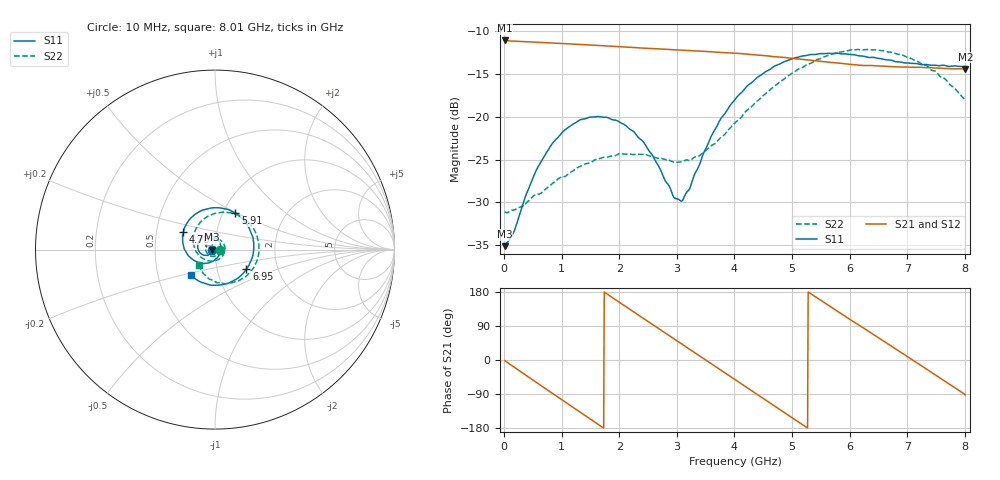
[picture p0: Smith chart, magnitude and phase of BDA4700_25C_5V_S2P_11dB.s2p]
!Agilent Technologies,E5071B,MY42404982,A.09.10
!Date: Mon Oct 20 13:31:35 2025
!Data & Calibration Information:
!Freq	S11:SOLT2(ON)	S21:SOLT2(ON)	S12:SOLT2(ON)	S22:SOLT2(ON)
# Hz S RI R 50
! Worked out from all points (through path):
!   801 points, 10 MHz to 8.01 GHz, reference 50 ohm
!   highest |S21| = -11.11 dB at 10 MHz (marker M1); lowest = -14.4 dB at 8.01 GHz (marker M2)
!   group delay of S21, straight-line fit = 281 ps
!   lowest |S11| = -35.1 dB at 10 MHz (marker M3), VSWR 1.04, Z = 48.3 - j0.111 ohm
!   |S11| at or under -10 dB: start of sweep to end of sweep
!   |S22| runs from -31.2 to -12.2 dB; largest |S21 - S12| = 0.002
!   S11 on the Smith chart (normalised r, x): 10 MHz: 0.97, -0.00; 4.78 GHz: 0.69, +0.14; 5.91 GHz: 1.14, +0.49; 6.95 GHz: 1.38, -0.31; 8.01 GHz: 0.74, -0.22
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1e7  -0.0175 -0.00115  0.2781 -0.00612  0.278 -0.00623  0.0279 -0.00149
1.6e8  -0.0186 -0.00972  0.2635 -0.0813  0.2634 -0.0815  0.0269 -0.00963
3.3e8  -0.024 -0.0199  0.2244 -0.157  0.2244 -0.1571  0.0222 -0.0205
7.2e8  -0.0507 -0.0327  0.0672 -0.2614  0.0672 -0.2615  -0.00319 -0.0376
1.02e9  -0.0784 -0.0227  -0.0763 -0.2557  -0.0765 -0.2558  -0.0304 -0.0325
1.35e9  -0.0962 0.00795  -0.2037 -0.1668  -0.2038 -0.167  -0.0516 -0.00399
1.94e9  -0.0649 0.0699  -0.2391 0.0933  -0.2391 0.0933  -0.0232 0.0547
2.33e9  -0.0151 0.0742  -0.1218 0.2207  -0.1219 0.2206  0.0235 0.0556
2.68e9  0.0222 0.0467  0.0287 0.2469  0.0286 0.2468  0.0527 0.0222
2.95e9  0.0326 0.00905  0.1375 0.2034  0.1374 0.2031  0.0528 -0.0124
3.09e9  0.0301 -0.0117  0.1824 0.1624  0.1816 0.1628  0.0454 -0.0306
3.54e9  -0.017 -0.0669  0.239 -0.0162  0.239 -0.0165  -0.00961 -0.0644
4.01e9  -0.1077 -0.0647  0.1454 -0.1838  0.1455 -0.1836  -0.0833 -0.0387
4.39e9  -0.1687 -0.00152  -0.00118 -0.2288  -0.00132 -0.2293  -0.1198 0.0284
4.78e9  -0.1758 0.1002  -0.1434 -0.1704  -0.1427 -0.171  -0.1046 0.1189
5.35e9  -0.065 0.2209  -0.211 0.0282  -0.2112 0.0275  0.0242 0.2055
5.91e9  0.1133 0.2027  -0.091 0.1823  -0.0912 0.182  0.1874 0.1497
6.3e9  0.1962 0.1051  0.0391 0.1949  0.0402 0.1941  0.2438 0.0332
6.68e9  0.2126 -0.0246  0.1482 0.1284  0.1486 0.1282  0.2214 -0.0872
6.95e9  0.1754 -0.1077  0.1884 0.0486  0.1887 0.0478  0.1676 -0.1522
7.48e9  0.0248 -0.1978  0.1505 -0.1197  0.1505 -0.1202  0.0115 -0.1843
8.01e9  -0.1345 -0.1426  -0.00565 -0.1896  -0.00546 -0.1898  -0.0911 -0.0846
